ORGANIZATION_BLOCK MAIN:OB1
TITLE= Inversione di Marcia di un M.A.T
// Simulatore: 01
// Versione: 1.0
// DATA: 26/02/2002
//
//***DESCRIZIONE***
// Il motore viene inserito tramite il pulsante SB2
// per il funzionamento in "Marcia Avanti", e SB3  per
// la "Marcia Indietro".
// Il Pulsante SB1  viene usato per arrestare la marcia
// del motore in qualsiasi momento.
// Il motore può essere commutato direttamente da uno all'altro
// senso di marcia senza che esso debba essere disinserito
// mediante il pulsante di arresto SB1.
//
// Per motivi di sicurezza un contatto NC del Relè Termico FR
// viene collegato, in hardware, a monte delle bobine dei contattori
// in modo da consentire la sicura diseccitazione dei contattori
// stessi in caso di intervento della protezione.
// Un contatto NC di RT viene però riportato anche su un ingresso
// del PLC per disattivare le uscite del PLC in caso
// di intervento dello stesso e segnalarne lo stato mediante la
// lampada di segnalazione HL1.
//
// Oltre all'interblocco hardware per impedire l'eccitazione
// contemporanea dei due contattori ( sempre indispensabile!) il
// programma ne effettua anche uno software  interrogando lo
// stato delle uscite dei contattori KM1 e KM2.
//

BEGIN
NETWORK 1 //Gestione Marcia Indietro Motore
//
LD I0.3
O Q0.0
A I0.1
AN I0.2
A I0.5
AN Q0.1
= Q0.0

NETWORK 2 //Gestione Marcia Avanti Motore
//
LD I0.2
O Q0.1
A I0.1
AN I0.3
A I0.5
AN Q0.0
= Q0.1

NETWORK 3 //Segnalazione motore fermo
//
LDN Q0.0
AN Q0.1
= Q0.2

NETWORK 4 //Segnalazione Marcia Avanti
//
LD Q0.1
= Q0.3

NETWORK 5 //Segnalazione Marcia indietro
//
LD Q0.0
= Q0.4

NETWORK 6 //Segalazione Relè Termico scattato
//
LDN I0.5
= Q0.5

END_ORGANIZATION_BLOCK

